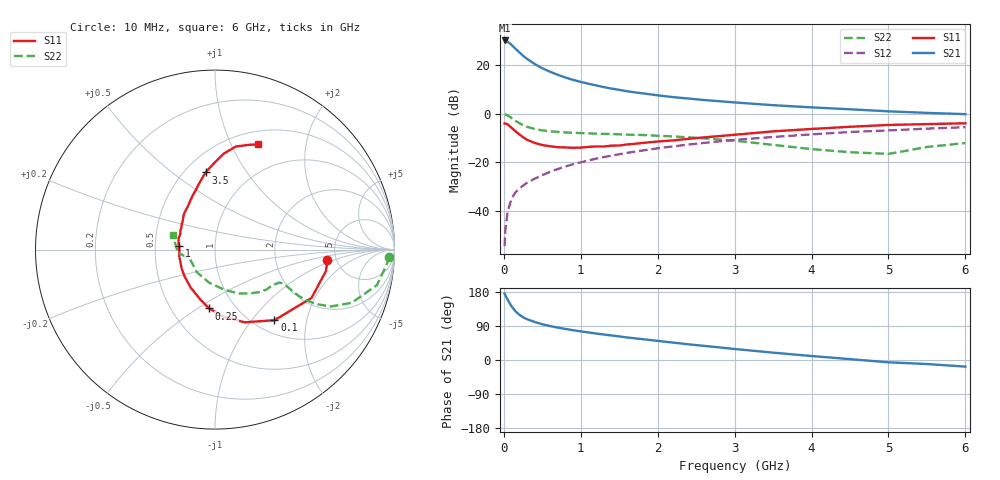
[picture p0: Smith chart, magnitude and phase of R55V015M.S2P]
! SIEMENS Small Signal Semiconductors
! BFR183
! Si NPN RF Bipolar Junction Transistor in SOT23
! VCE = 5 V  IC = 15 mA
! Common Emitter S-Parameters:  May  1996
# GHz  S  MA  R  50
!  f  S11  S21  S12  S22
! GHz  MAG  ANG  MAG  ANG  MAG  ANG  MAG  ANG
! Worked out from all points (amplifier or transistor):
!   36 points, 10 MHz to 6 GHz, reference 50 ohm
!   highest |S21| = 30.1 dB at 10 MHz (marker M1)
!   |S21| within 3 dB of that: start of sweep to 138.7 MHz
!   unconditionally stable (mu >= 1): 673.9 MHz to 2.49 GHz
!   at 250 MHz: K = 0.73, MSG = 26.7 dB, |S12| = -29.6 dB
!   at 1.4 GHz: K = 1.05, MAG = 12.5 dB, |S12| = -17.2 dB
!   at 6 GHz: K = 0.89, MSG = 2.7 dB, |S12| = -5.6 dB
!   S11 on the Smith chart (normalised r, x): 10 MHz: 4.23, -0.83; 100 MHz: 1.22, -1.31; 250 MHz: 0.76, -0.56; 1 GHz: 0.67, +0.03; 3.5 GHz: 0.63, +0.67; 6 GHz: 0.65, +1.28
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0.01  0.6295 -5.4  31.89 175.3  0.0019 86.9  0.9704 -2.4
0.02  0.6294 -11.0  31.63 170.8  0.0042 89.3  0.9589 -5.2
0.05  0.6016 -26.6  30.1 158.8  0.0099 77.3  0.9235 -12.4
0.1  0.5143 -49.9  26.01 141.8  0.0178 72.0  0.8169 -21.3
0.15  0.4374 -67.9  21.67 128.7  0.0241 66.9  0.7163 -26.3
0.2  0.3763 -82.6  18.24 119.7  0.0288 66.1  0.6391 -28.3
0.25  0.3293 -95.7  15.49 112.8  0.0333 66.1  0.5788 -29.0
0.3  0.2915 -105.9  13.41 107.7  0.0381 66.7  0.5385 -29.0
0.4  0.2508 -122.9  10.51 100.4  0.0461 67.6  0.486 -28.1
0.5  0.2266 -137.9  8.551 94.3  0.0547 68.2  0.454 -27.2
0.6  0.2144 -149.6  7.257 89.6  0.0637 69.0  0.4344 -26.7
0.7  0.2047 -160.5  6.29 85.6  0.0729 69.2  0.4222 -26.7
0.8  0.2027 -169.4  5.524 81.9  0.082 69.1  0.4118 -26.8
1  0.2011 174.7  4.492 75.5  0.1001 68.3  0.3994 -27.6
1.1  0.2076 169.0  4.12 72.8  0.1095 68.2  0.394 -28.7
1.3  0.2119 156.0  3.511 67.2  0.1285 66.7  0.3845 -30.4
1.6  0.2329 142.8  2.895 59.5  0.1565 64.4  0.3706 -34.3
2.2  0.2825 122.8  2.188 45.9  0.2131 58.6  0.3416 -43.9
3.5  0.4333 97.0  1.494 19.4  0.3321 43.0  0.2287 -77.2
4.5  0.5377 84.7  1.23 2.3  0.4201 30.6  0.1616 -128.9
5.5  0.611 72.6  1.038 -10.6  0.4931 18.9  0.2068 -175.2
6  0.6347 67.6  0.978 -17.5  0.5276 11.4  0.2495 161.2
